FUNCTION_BLOCK FB103
TITLE =Restore
//*****************************************************************************
//* maxon motor ag
//* R&D
//* all rights reserved
//*****************************************************************************
//* Summary:  Restore all system parameters
//*
//* Remarks:
//*
//* Created under: STEP7 REV5.2+SP1
//*****************************************************************************
//* History:
//* 18.05.2004 | INA   first release
//*
//*
//*****************************************************************************
//

AUTHOR:INA
FAMILY:Utilitie
NAME:Restore
VERSION:00.01


VAR_INPUT

Write : BOOL //A rising edge start the command

  NodeID : BYTE //Adress of the maxon device

END_VAR
VAR_OUTPUT
  Done : BOOL //Data valid flag is TRUE if data were available

  Err : BOOL //Error flag is TRUE if an Error has occured, see ErrNo for more details

  ErrNo : DINT //Contains detailed error information

END_VAR
VAR
  xEdgeMerker : BOOL //Edge Merker

  xEdgeFlag : BOOL //Edge Flag

  xStep : INT
  xRestoreAllParameters : DWORD  := DW#16#64616F6C
END_VAR

BEGIN

NETWORK
TITLE = Activate the service function
//

// SDO Write "Restore"

       U    #Write
       FP   #xEdgeFlag                   // recognize a positiv edge of the Read signal
       =    #xEdgeMerker                 // and set the xEdgeMerker for one cycle to true

       L    #xStep
       L    0
       ==I
       U    #xEdgeMerker
       SPB  nstp                         // iStep = 1 -> fnc1

       L    #xStep                       // jump list
       SPL  List
       SPA  rdef
       SPA  fnc1
       SPA  fncE
List  :SPA  rdef

rdef  :NOP  0
       R    #Done                        // reset Done
       R    #Err
       L    0
       T    #xStep                       // iStep = 0
       SPA  end

fnc1  :NOP  0
       CALL FC16
         NodeID:=#NodeID
         Index:=DW#16#00001011
         SubIndex:=DW#16#00000001
         ValueIn:=#xRestoreAllParameters
         RET_VAL:=#Done
         Err:=#Err
         ErrNo:=#ErrNo

fncE  :NOP  0
       L    0
       T    #xStep
       SPA  end

nstp  :NOP  0
       L    #xStep
       INC            1
       T    #xStep

end   :NOP  0
END_FUNCTION_BLOCK
